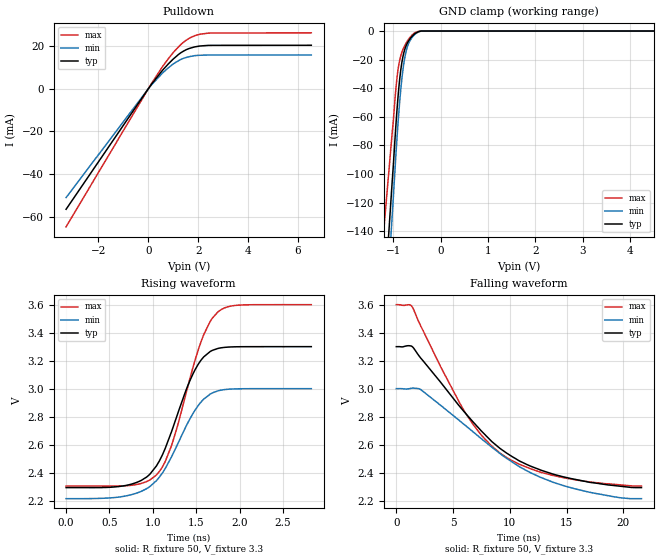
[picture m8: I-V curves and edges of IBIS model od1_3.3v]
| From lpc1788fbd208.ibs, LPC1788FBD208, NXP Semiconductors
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[Model]   od1_3.3v
Model_type I/O_open_drain
Vinl=8.000E-01
Vinh=2.000E+00
Vref=3.300E+00
Rref=2.000E+03
Cref=0.000E+00
Vmeas=1.650E+00
C_comp   1.240E-12   1.180E-12   1.300E-12
[Voltage Range]   3.300E+00   3.000E+00   3.600E+00
[POWER Clamp Reference]   3.300E+00   3.000E+00   3.600E+00
[GND Clamp Reference]   0.000E+00   0.000E+00   0.000E+00
[Pullup Reference]   3.300E+00   3.000E+00   3.600E+00
[Pulldown Reference]   0.000E+00   0.000E+00   0.000E+00
[Temperature Range]   25   85   -40
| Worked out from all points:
|   slope of the pulldown table from 0 to 0.495 V, typ, clamps not added: 65.7 ohm
|   GND clamp passes 1 mA (typ) near -0.51 V on its own axis
|   rising waveform, R_fixture 50, V_fixture 3.3: 20-80 % time 373ps typ, 403ps min, 362ps max; typ from 2.29 V to 3.3 V
|   falling waveform, R_fixture 50, V_fixture 3.3: 20-80 % time 7.24ns typ, 8.09ns min, 5.99ns max; typ from 3.3 V to 2.29 V
[GND Clamp]
-3.3V     -1.237A    -1.348A    -943.1mA
-1.025V   -104mA     -127.6mA   -70.1mA
-944.8mV  -63.91mA   -84.53mA   -38.83mA
-904.9mV  -46.41mA   -64.86mA   -27.25mA
-864.9mV  -32.54mA   -47.93mA   -19.82mA
-805.1mV  -18.69mA   -28.34mA   -13.29mA
-765.1mV  -13.22mA   -19.31mA   -10.38mA
-705.3mV  -8.281mA   -10.85mA   -6.894mA
-625.4mV  -4.434mA   -5.339mA   -3.493mA
-525.6mV  -1.357mA   -1.755mA   -822.7uA
-405.9mV  0A         0A         0A
6.6V      0A         0A         0A
[Pulldown]
-3.3V     -56.5mA    -51.02mA   -64.74mA
133mV     2.157mA    1.865mA    2.546mA
552.2mV   8.383mA    7.138mA    10.03mA
791.7mV   11.49mA    9.679mA    13.86mA
1.011V    14.03mA    11.69mA    17.12mA
1.41V     17.6mA     14.25mA    21.79mA
1.65V     18.89mA    15.04mA    23.71mA
1.869V    19.61mA    15.52mA    24.88mA
2.389V    20.29mA    15.78mA    26.03mA
6.54V     20.37mA    15.82mA    26.19mA
[Rising Waveform]
R_fixture = 50
V_fixture = 3.3
V_fixture_min = 3
V_fixture_max = 3.6
0s        2.293V     2.214V     2.304V
725ps     2.314V     2.239V     2.308V
925ps     2.368V     2.285V     2.336V
1.041ns   2.448V     2.343V     2.384V
1.214ns   2.692V     2.512V     2.592V
1.487ns   3.136V     2.848V     3.206V
1.586ns   3.227V     2.925V     3.386V
1.76ns    3.289V     2.986V     3.553V
1.983ns   3.299V     2.999V     3.596V
2.825ns   3.3V       3V         3.6V
[Falling Waveform]
R_fixture = 50
V_fixture = 3.3
V_fixture_min = 3
V_fixture_max = 3.6
0s        3.3V       3V         3.6V
1.373ns   3.302V     3.003V     3.588V
2.147ns   3.219V     2.994V     3.449V
5.968ns   2.836V     2.745V     2.843V
7.541ns   2.694V     2.639V     2.663V
9.139ns   2.573V     2.536V     2.54V
11.5ns    2.458V     2.413V     2.438V
14.66ns   2.371V     2.309V     2.366V
19.05ns   2.309V     2.229V     2.317V
21.6ns    2.293V     2.214V     2.304V
[Ramp]
dV/dt_r   6.0392E-01/3.7240E-10   4.7144E-01/4.0290E-10   7.7735E-01/3.5950E-10
dV/dt_f   6.0392E-01/7.2206E-09   4.7144E-01/8.0847E-09   7.7735E-01/5.9653E-09
R_load = 50
